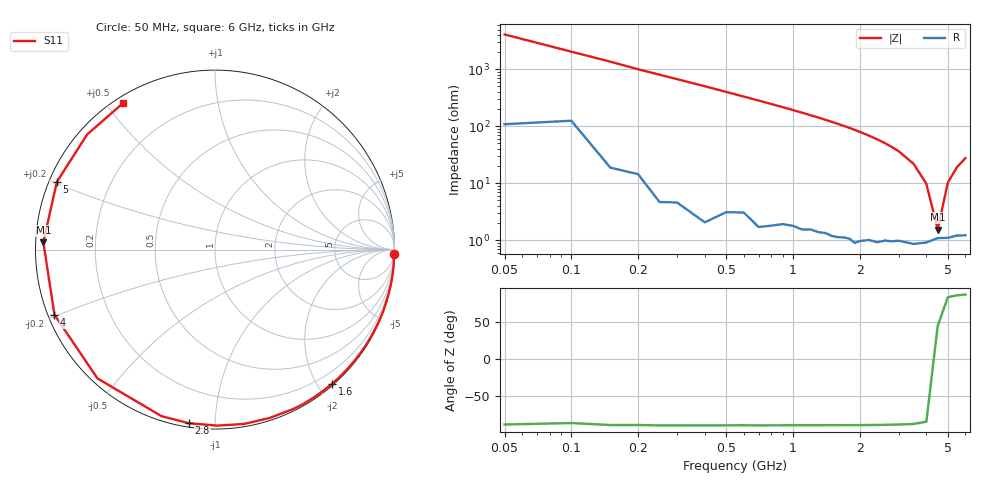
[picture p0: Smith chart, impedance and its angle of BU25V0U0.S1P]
! Infineon Technologies  Discrete & RF Semiconductors
! BB 833
! Si Tuning Diode in SOD323
! VR = 25 V
! S-Parameters:  June  1999
# GHz  S  MA  R  50
!  f  S11
! GHz  MAG  ANG
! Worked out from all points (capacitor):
!   34 points, 50 MHz to 6 GHz, reference 50 ohm
!   read as one part to ground: C = 778 fF near 50 MHz
!   lowest |Z| = 1.54 ohm at 4.5 GHz (marker M1)
!   series resonance near 4.45 GHz, so ESL is about 1.6 nH
!   S11 on the Smith chart (normalised r, x): 50 MHz: 2, -82; 1.6 GHz: 0.02, -2.20; 2.8 GHz: 0.02, -0.86; 4 GHz: 0.02, -0.20; 5 GHz: 0.02, +0.21; 6 GHz: 0.02, +0.55
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0.05  0.9993 -1.4
0.25  0.9993 -7.1
0.4  0.9992 -11.3
0.5  0.9981 -14.2
0.7  0.9979 -20.0
0.8  0.9971 -23.0
1  0.9955 -29.1
1.1  0.9953 -32.2
1.2  0.9943 -35.4
1.3  0.9939 -38.6
1.4  0.9931 -42.0
1.5  0.9929 -45.4
1.6  0.9923 -48.9
1.7  0.9913 -52.5
1.8  0.9906 -56.2
1.9  0.991 -60.0
2  0.9892 -63.9
2.2  0.9861 -72.0
2.4  0.9847 -80.5
2.6  0.9807 -89.2
2.8  0.9783 -98.5
3  0.9747 -107.8
3.5  0.9715 -132.4
4  0.9654 -157.9
4.5  0.9574 177.5
5  0.9585 156.8
5.5  0.9586 138.0
6  0.9632 122.2
